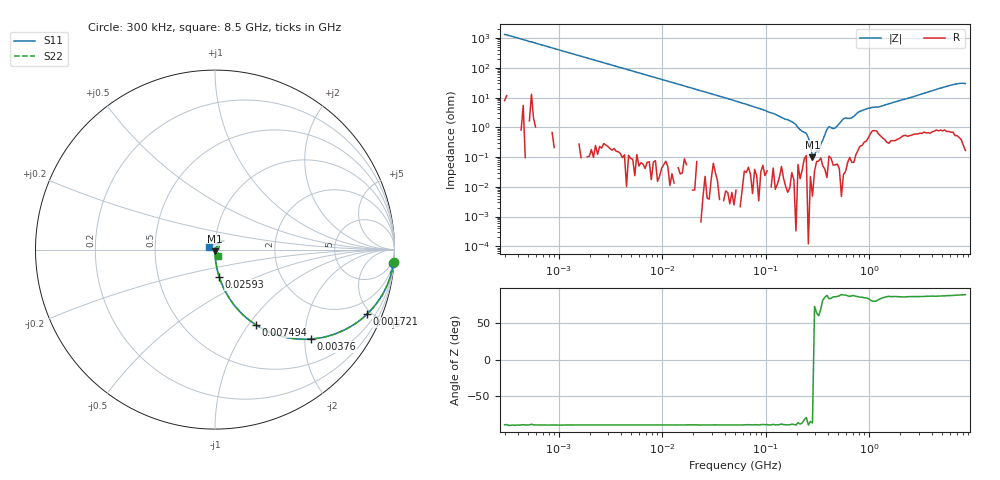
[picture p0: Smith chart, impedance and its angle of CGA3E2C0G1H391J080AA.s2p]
! S-parameter Generated by TDK Corporation
! Copyright(C) 2015 TDK Corporation.
! All Rights Reserved.
! TDK P/N: CGA3E2C0G1H391J080AA (Multilayer Ceramic Chip Capacitors)
! Property: C=390pF
! Size(LxWxT): 1.6x0.8x0.8mm, 0.063x0.031x0.031inches
! Model Type: s2p (Touchstone File Format Version 1.0)
! Frequency: DC=Yes Start=0.3MHz Stop=8500MHz 225points Log-sweep
! Note:
! Model Generated on Jun. 23, 2015
! Hash(MD5):
! Port Assignments:
!  1 ---| |--- 2
! Applicable Conditions:
!  Temperature = 25 degC
!  DC Bias Voltage = 0 V
!  Small Signal Operation
! Terms and conditions regarding TDK Simulation Models
! (1)This simulation model is being provided solely for informational purposes. Please refer to the specifications of the products in terms of detailed characteristics of such products.
! (2)In no event shall TDK Corporation of any of its subsidiaries be liable for any loss or damage arising, directly or indirectly,
!  From any information contained in this simulation model, including, but not limited to loss or damages arising from any inaccuracies, omissions or errors in connection with such information.
! (3)Any and all copyrights on this simulation model are owned by TDK Corporation.
!  Duplication or redistribution of this simulation model without prior written permission from TDK Corporation is prohibited.
! (4)This simulation model is subject to any modification or change without any prior notice.
! (5)Neither TDK Corporation nor any of its subsidiaries shall make any warranty, express or implied,
!  Including but not limited to the correctness, implied warranties of merchantability and fitness for a particular purpose with respect to this simulation models.
! (6)The use of this simulation model shall be deemed to have consented to the terms and conditions hereof.
# MHz S MA R 50
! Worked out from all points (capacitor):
!   224 points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, 300 kHz to 8.5 GHz, reference 50 ohm
!   read as one part in series: C = 393 pF near 314.1 kHz
!   lowest |Z| = 98.9 mohm at 283.1 MHz (marker M1)
!   series resonance near 289.3 MHz, so ESL is about 770 pH
!   S11 on the Smith chart (normalised r, x): 300 kHz: 1, -27; 1.721 MHz: 1.01, -4.70; 3.76 MHz: 1.00, -2.15; 7.494 MHz: 1.00, -1.08; 25.93 MHz: 1.00, -0.31; 8.5 GHz: 0.93, +0.03
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0.3  0.9967 -4.2  0.07513 85.6  0.07511 85.7  0.9969 -3.9
1.72111  0.9196 -23.1  0.392 67.0  0.3914 66.9  0.9198 -23.1
3.760292  0.7318 -42.9  0.6802 47.1  0.6807 47.1  0.7323 -42.9
7.493824  0.4751 -61.6  0.8799 28.3  0.8784 28.4  0.4749 -61.8
9.430415  0.3943 -66.8  0.919 23.1  0.919 23.2  0.3943 -66.8
25.92811  0.154 -81.2  0.9881 8.7  0.9874 8.8  0.1539 -81.3
51.67171  0.07734 -85.5  0.9968 4.3  0.997 4.2  0.07736 -85.9
283.1228  0.009409 -89.2  0.9999 -0.4  0.9999 -0.5  0.009444 -91.2
340.2802  0.007045 -81.3  0.9983 -0.7  0.9985 -0.7  0.006019 -95.8
408.9767  0.002593 -75.6  0.9982 -1.4  0.9984 -1.4  0.003327 -88.0
448.3627  0.003075 -62.9  0.9991 -1.1  0.9995 -1.2  0.002109 -109.7
514.6664  0.0008398 0.0  0.9995 -1.6  0.9995 -1.5  0.0006958 -105.9
564.2308  0.001397 30.8  0.9998 -2.2  0.9992 -2.1  0.00187 121.9
618.5683  0.002588 60.3  0.9999 -2.2  0.9984 -2.2  0.001797 100.4
979.5854  0.009408 68.8  0.9957 -4.4  0.9955 -4.5  0.01131 53.4
1290.729  0.005441 41.3  0.9945 -5.6  0.9948 -5.5  0.007697 32.6
1551.304  0.006797 72.3  0.997 -6.8  0.997 -6.7  0.007763 47.7
2456.696  0.01098 59.8  0.995 -10.9  0.994 -10.6  0.01087 38.7
5884.306  0.06333 48.7  0.9908 -26.1  0.9897 -26.0  0.06219 65.6
7404.957  0.06068 49.4  0.9915 -32.5  0.9908 -32.6  0.0575 60.3
8118.083  0.02928 84.8  0.9918 -35.5  0.9917 -35.4  0.02276 21.3
8500  0.03839 155.4  0.9912 -37.1  0.9934 -36.9  0.03946 -65.4
